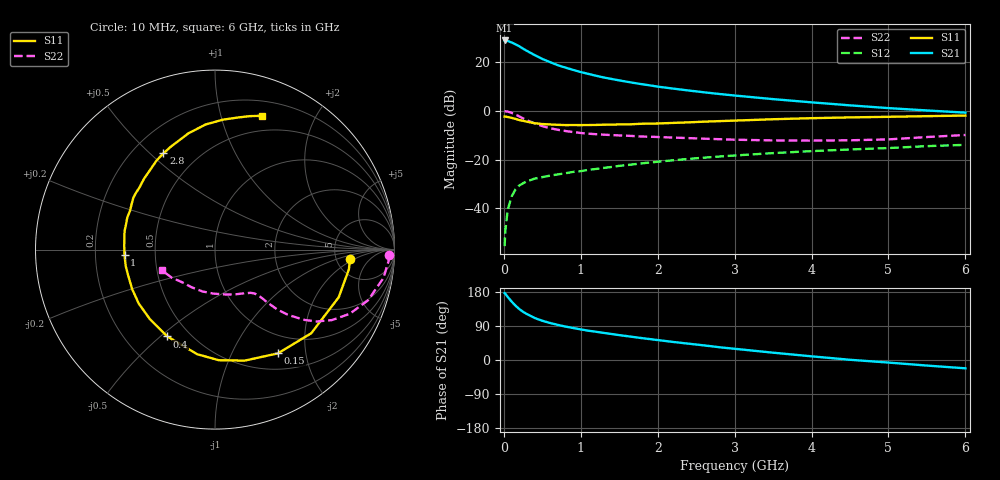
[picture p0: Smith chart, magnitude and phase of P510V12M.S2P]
! SIEMENS Small Signal Semiconductors
! BFP183
! Si NPN RF Bipolar Junction Transistor in SOT143
! VCE = 10 V  IC = 12 mA
! Common Emitter S-Parameters:  March  1996
# GHz  S  MA  R  50
!  f  S11  S21  S12  S22
! GHz  MAG  ANG  MAG  ANG  MAG  ANG  MAG  ANG
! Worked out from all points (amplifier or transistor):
!   36 points, 10 MHz to 6 GHz, reference 50 ohm
!   highest |S21| = 28.6 dB at 10 MHz (marker M1)
!   |S21| within 3 dB of that: start of sweep to 231.4 MHz
!   unconditionally stable (mu >= 1): 1.196 GHz to 5.853 GHz
!   at 250 MHz: K = 0.33, MSG = 27.5 dB, |S12| = -29.7 dB
!   at 1.4 GHz: K = 1.06, MAG = 16.5 dB, |S12| = -23.0 dB
!   at 6 GHz: K = 0.98, MSG = 6.6 dB, |S12| = -14.0 dB
!   S11 on the Smith chart (normalised r, x): 10 MHz: 6.72, -1.64; 150 MHz: 0.72, -1.53; 400 MHz: 0.38, -0.53; 1 GHz: 0.33, -0.03; 2.8 GHz: 0.32, +0.55; 6 GHz: 0.34, +1.36
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0.01  0.7539 -4.0  27.02 176.6  0.0017 68.7  0.9725 -1.8
0.02  0.754 -8.4  26.85 174.5  0.0036 77.3  0.9686 -3.9
0.05  0.7387 -21.1  26.4 166.5  0.0093 79.2  0.9521 -9.5
0.1  0.7104 -41.0  24.62 154.4  0.0174 69.6  0.8987 -18.3
0.15  0.676 -58.8  22.59 143.7  0.0243 62.3  0.8314 -25.5
0.2  0.6403 -75.0  20.55 134.6  0.0294 56.9  0.7602 -31.1
0.25  0.6167 -88.0  18.33 127.1  0.0327 52.9  0.6932 -35.3
0.3  0.5912 -99.7  16.55 121.2  0.0359 50.0  0.6355 -38.1
0.4  0.5519 -118.8  13.59 110.9  0.0407 46.4  0.546 -41.8
0.5  0.5307 -133.2  11.33 103.5  0.0437 43.5  0.4812 -43.9
0.6  0.5203 -144.8  9.772 97.7  0.0468 43.4  0.4363 -44.8
0.7  0.5114 -154.4  8.457 92.7  0.0496 42.6  0.4053 -45.4
0.8  0.505 -162.4  7.542 88.3  0.0524 42.5  0.3824 -45.8
1  0.505 -176.4  6.11 80.7  0.0579 43.6  0.3483 -46.8
1.1  0.5062 177.9  5.603 77.3  0.0616 43.5  0.337 -47.4
1.5  0.5207 159.8  4.132 65.6  0.0742 43.9  0.3105 -50.9
2.2  0.5595 134.8  2.808 47.7  0.0965 41.9  0.2807 -61.6
2.8  0.6084 118.2  2.181 33.7  0.1151 38.4  0.2603 -74.2
3.5  0.6648 102.8  1.712 19.3  0.1352 33.6  0.2455 -91.8
4.5  0.7249 86.6  1.277 0.6  0.1605 25.9  0.2471 -122.0
5.5  0.7684 75.4  1.005 -14.7  0.1877 19.3  0.2879 -147.2
6  0.7909 70.5  0.906 -22.0  0.1995 15.0  0.3171 -158.8
